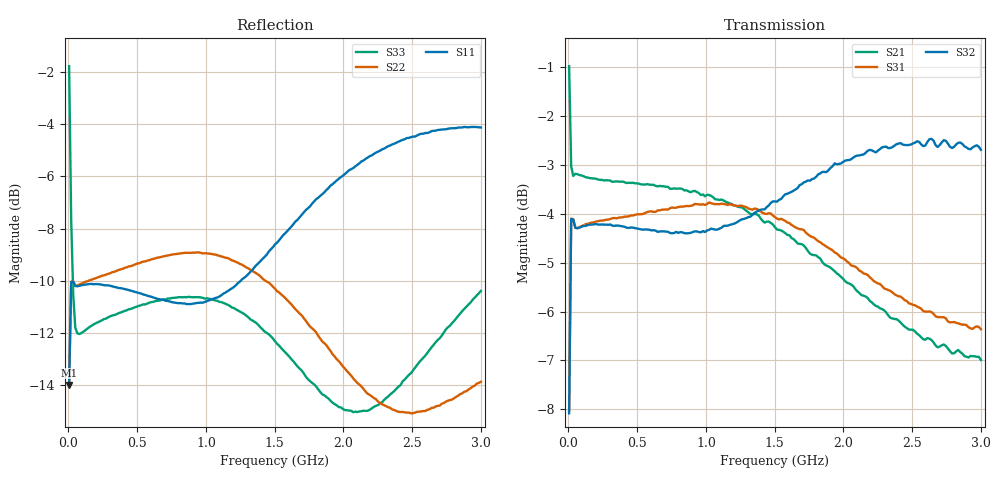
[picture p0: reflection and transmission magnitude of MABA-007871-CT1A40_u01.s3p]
#	MHz	S	RI	R	50
!FREQ	R1	I1	R2	I2	R3	I3
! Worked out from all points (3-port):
!   201 points, 5 MHz to 3 GHz, reference 50 ohm
!   strongest paths, dB at 5 MHz, 753.8 MHz, 1.502 GHz, 2.251 GHz, 3 GHz:
!     S32: -8.1, -4.4, -3.7, -2.7, -2.7
!     S31: -8.0, -3.9, -4.1, -5.4, -6.4
!     S21: -1.0, -3.5, -4.3, -5.9, -7.0
!   lowest |S11| = -14.0 dB at 5 MHz (marker M1), VSWR 1.50, Z = 60.5 + j19.8 ohm
!   |S11| at or under -10 dB: start of sweep to 1.253 GHz
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5  0.1233 0.1572  0.8781 -0.1631  -0.2444 -0.3126
   0.8789 -0.1624  0.1201 0.1579  0.2426 0.3135
   -0.2444 -0.3126  0.2394 0.3132  -0.515 0.6305
19.975  0.304 0.0807  0.6977 -0.1063  -0.6016 -0.1651
        0.6976 -0.1068  0.3016 0.0908  0.5982 0.1751
        -0.6016 -0.1651  0.5984 0.1748  0.2045 0.3607
34.95  0.3139 0.0236  0.6863 -0.0696  -0.6205 -0.0559
       0.6863 -0.0699  0.3126 0.0418  0.6182 0.0744
       -0.6205 -0.0559  0.6183 0.0742  0.246 0.1666
813.65  0.00111 -0.2866  0.3863 -0.549  -0.3817 0.5158
        0.3896 -0.5448  0.3488 -0.0749  0.594 -0.1121
        -0.3817 0.5158  0.5936 -0.1135  0.2941 -0.00854
1143.1  -0.2241 -0.1999  0.1224 -0.6385  -0.1475 0.6282
        0.1335 -0.6354  0.3204 -0.141  0.5968 -0.1461
        -0.1475 0.6282  0.5958 -0.1465  0.2814 -0.0494
1502.5  -0.366 0.0612  -0.1752 -0.5783  0.1284 0.6127
        -0.1625 -0.5894  0.2453 -0.1819  0.6209 -0.2027
        0.1284 0.6127  0.6171 -0.2029  0.2319 -0.0698
1802  -0.3213 0.3194  -0.3552 -0.4278  0.3064 0.5089
      -0.3534 -0.4499  0.183 -0.1731  0.6383 -0.2787
      0.3064 0.5089  0.631 -0.2756  0.1922 -0.0491
2236.275  -0.0362 0.555  -0.4601 -0.153  0.4426 0.304
          -0.4804 -0.1645  0.1429 -0.1218  0.6071 -0.4255
          0.4426 0.304  0.5982 -0.4174  0.1816 0.014
2565.725  0.2303 0.5589  -0.4496 0.0349  0.478 0.1615
          -0.4698 0.0423  0.1507 -0.0945  0.5379 -0.5342
          0.478 0.1615  0.5307 -0.5202  0.2168 0.0525
3000  0.4961 0.3744  -0.3628 0.2395  0.4807 -0.00587
      -0.3644 0.259  0.1786 -0.0958  0.3997 -0.6365
      0.4807 -0.00587  0.3958 -0.618  0.2956 0.0635
